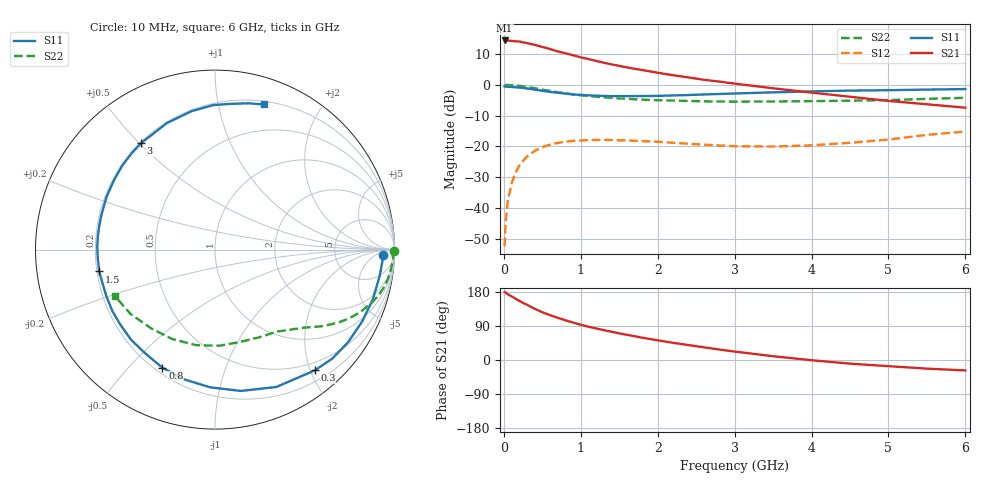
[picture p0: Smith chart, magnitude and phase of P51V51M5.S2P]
! SIEMENS Small Signal Semiconductors
! BFP183
! Si NPN RF Bipolar Junction Transistor in SOT143
! VCE = 1.5 V  IC = 1.5 mA
! Common Emitter S-Parameters:  March  1996
# GHz  S  MA  R  50
!  f  S11  S21  S12  S22
! GHz  MAG  ANG  MAG  ANG  MAG  ANG  MAG  ANG
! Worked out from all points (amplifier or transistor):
!   36 points, 10 MHz to 6 GHz, reference 50 ohm
!   highest |S21| = 14.4 dB at 10 MHz (marker M1)
!   |S21| within 3 dB of that: start of sweep to 628.8 MHz
!   unconditionally stable (mu >= 1): 2.223 GHz to end of sweep
!   at 250 MHz: K = 0.11, MSG = 19.2 dB, |S12| = -24.7 dB
!   at 1.4 GHz: K = 0.62, MSG = 12.3 dB, |S12| = -17.9 dB
!   at 6 GHz: K = 1.05, MAG = 2.6 dB, |S12| = -15.2 dB
!   S11 on the Smith chart (normalised r, x): 10 MHz: 26, -12; 300 MHz: 0.37, -2.07; 800 MHz: 0.23, -0.63; 1.5 GHz: 0.21, -0.09; 3 GHz: 0.20, +0.51; 6 GHz: 0.23, +1.37
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0.01  0.9372 -1.7  5.25 179.1  0.0024 85.5  0.9993 -0.6
0.02  0.9358 -3.5  5.221 178.2  0.0051 85.2  0.9903 -1.3
0.05  0.9295 -8.9  5.237 174.0  0.0129 87.3  0.9937 -3.3
0.1  0.9221 -17.4  5.171 168.1  0.0247 78.6  0.9854 -6.7
0.2  0.9034 -34.8  5.046 156.3  0.0483 69.7  0.9624 -12.9
0.25  0.8921 -42.9  4.898 150.7  0.0583 65.4  0.9446 -15.9
0.3  0.873 -50.4  4.749 146.0  0.0682 61.1  0.9232 -18.5
0.4  0.8383 -65.9  4.459 135.3  0.0844 52.7  0.8814 -23.3
0.5  0.8006 -79.6  4.118 126.1  0.0971 45.4  0.8362 -27.5
0.6  0.7678 -92.0  3.815 118.4  0.1068 39.2  0.7954 -30.8
0.7  0.7432 -103.3  3.484 111.3  0.1139 34.1  0.7596 -33.5
0.8  0.7201 -114.0  3.253 104.7  0.1192 29.4  0.7293 -35.9
1  0.6864 -132.8  2.796 93.1  0.1247 21.5  0.6754 -39.9
1.1  0.6731 -141.6  2.619 87.8  0.1268 18.5  0.6557 -41.6
1.5  0.6565 -169.3  2.031 70.3  0.1256 9.1  0.6011 -47.9
1.8  0.657 173.3  1.733 58.8  0.1219 4.8  0.5741 -52.6
2.2  0.6719 154.2  1.43 45.3  0.1147 1.4  0.5548 -59.5
3  0.7224 124.7  1.046 22.3  0.1008 3.2  0.5329 -75.9
3.5  0.7543 110.8  0.878 10.0  0.0995 8.8  0.5361 -87.4
4.5  0.8055 90.6  0.64 -9.6  0.1145 19.5  0.5525 -115.6
5.5  0.8363 77.1  0.483 -22.8  0.154 22.1  0.5915 -142.6
6  0.8531 71.4  0.425 -27.5  0.1742 19.0  0.6156 -155.2
